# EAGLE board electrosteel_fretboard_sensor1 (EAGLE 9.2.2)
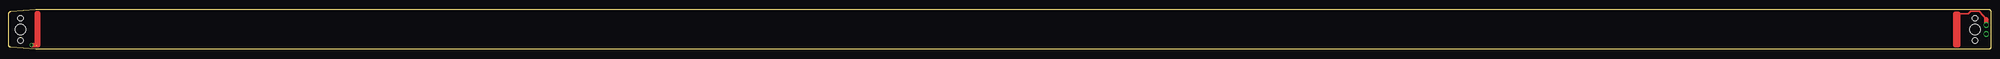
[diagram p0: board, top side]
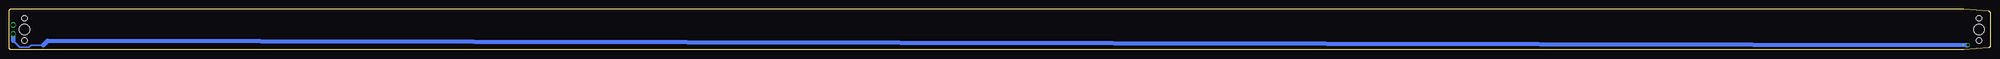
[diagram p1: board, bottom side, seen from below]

Size 562.99 x 11.43 mm. Coordinates in mm from the lower left corner, seen from the top.
Outline: 0.58,10.84 7.72,11.43 arc-5 7.77,11.43 562.36,11.43 arc-90 562.99,10.79 562.99,0.64 arc-90 562.36,0 7.65,0 arc-5 7.59,0 0.58,0.59 arc-85 0,1.22 0,10.21 arc-85 0.58,10.84
Copper layers (1*16): Top 0.035mm / dielectric 1.5mm / Bottom 0.035mm
Design rules "default *": minimum track width 10mil, minimum drill 24mil, track to track 8mil, track to pad 8mil, pad to pad 8mil, via to via 8mil, smd to smd 8mil, copper to edge 40mil, drill to drill 8mil, minimum pad ring 2mil, minimum via ring 8mil, stop-mask expansion 4mil, vias tented up to drill 0mil, thermal gap 10mil
Holes 3.05 mm at 558.55,5.71 3.3,5.71
Holes 1.52 mm at 558.55,8.89 558.55,2.54 3.3,8.89 3.3,2.54

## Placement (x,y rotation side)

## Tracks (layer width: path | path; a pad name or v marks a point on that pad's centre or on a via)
N$1  (via drill 1.02)
  Top 0.406: 561.72,8.64 559.76,10.79 557.28,10.79 556.64,10.16 553.85,10.16
  Top 1.27: 552.96,10.16 553.72,10.16 553.72,1.27 552.96,1.27 552.96,10.03 | 561.72,8.64 v561.72,6.99
S$26  (via drill 0.65, 1.02)  (1 unrouted)
  Top 1.27: v6.48,1.27 7.75,1.27 | 7.87,1.27 7.87,10.29 8.38,10.29 8.38,1.14 7.75,1.14
  Bottom 0.406: 561.72,2.54 559.82,0.64 557.28,0.64 556.64,1.27 553.21,1.27
  Bottom 1.27: 553.21,1.27 551.95,2.54 7.11,1.27 v6.48,1.27 | 561.72,2.54 v561.72,4.45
